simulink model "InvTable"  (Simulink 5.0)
settings: Solver=FixedStepDiscrete  StartTime=0.0  StopTime=inf  FixedStep=samplePeriod  RelTol=1e-3
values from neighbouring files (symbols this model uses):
  a0 = zeros(1, nAct)    [initialize.m]    (also in quake.m = 0; rspect.m = 1)
  azMask = zeros(nAcc, 1)    [initialize.m]
  bal = [[ 1  1  1  1  0  0  0  0  0  0  0  0]    [initialize.m]
  cmap = jet    [initialize.m]    (also in tableAnimation.m = self.cmap)
  ea_t = zeros(3, nAcc)    [initialize.m]
  faces = nAct               			+ [ 1  2  3  4    [initialize.m]    (also in tableAnimation.m = self.faces)
  flowCanon = 63090.2    [initialize.m]
  fmax = zeros(nAct, 1)    [initialize.m]
  gasConstant = 1.8    [initialize.m]
  gee = 1.0    (= 1)    [initialize.m]    (also in accelA2T.m = h(24); accelT2A.m = h(24); Test.m)
  iactParamsX = [actParamsX, dfGain, solver]    [initialize.m]
  iactParamsY = [actParamsY, dfGain, solver]    [initialize.m]
  iactParamsZ = [actParamsZ, dfGain, solver]    [initialize.m]
  inertia = [Ixx 0 0; 0 Iyy 0; 0 0 Izz]    [initialize.m]
  inertiaCanon = 0.1130    (= 0.113)    [initialize.m]
  linAccelCanon = 9800.0    (= 9800)    [initialize.m]    (also in accelA2T.m = h(19); accelT2A.m = h(19); Test.m)
  lines = nAct               			+ [ 1  2  3  4  1    				5  6  7  8  5    				9 10 11 12  9    				0  2  6 10       				0  3  7 11       				0  4  8 12  0];  	lines(find(lines==nAct)) = 0    [initialize.m]    (also in tableAnimation.m = self.lines; viewer.m = 1)
  linVelocCanon = 1000.0    (= 1000)    [initialize.m]    (also in Test.m)
  mass = [massX massY massZ]'    [initialize.m]
  massCanon = 0.4535924e-06    (= 4.535924e-07)    [initialize.m]
  maxDispl = [maxDisplX  			maxDisplY  			maxDisplZ  			maxDisplZ * linVelocCanon / rollRadius  * 180/pi  			maxDisplZ * linVelocCanon / pitchRadius * 180/pi  			min(maxDisplX, maxDisplY) * linVelocCanon / yawRadius * 180/pi]    [initialize.m]
  maxOilVolume = volume * (1 - (precharge/supplyPress)^(1/gasConstant))    (= 32.2704137442)    [initialize.m]
  maxVeloc = [maxVelocX  			maxVelocY  			maxVelocZ  			maxVelocZ * linVelocCanon / rollRadius  * 180/pi  			maxVelocZ * linVelocCanon / pitchRadius * 180/pi  			min(maxVelocX, maxVelocY) * linVelocCanon / yawRadius * 180/pi]    [initialize.m]
  minDispl = -maxDispl    [initialize.m]
  minVeloc = -maxVeloc    [initialize.m]
  nAct = size(rt_t, 2)    [initialize.m]    (also in tableAnimation.m = self.nAct)
  precharge = 2000    [initialize.m]
  pumpFlow = 1e10    (= 10000000000)    [initialize.m]
  ra_t = [  -20.0   -20.0   -92.0 -2590.0  2590.0   -62.0 -2133.0 -2133.0  2133.0  2133.0   -62.0    [initialize.m]    (also in accelA2T.m = [-h9   -h9 -h15 -h10  h10 -h14 -h12 -h12  h12  h12 -h16; accelT2A.m = [-h9   -h9 -h15 -h10  h10 -h14 -h12 -h12  h12  h12 -h16)
  rb_w = [-5692.1 -5692.1  5692.1  5692.1 -2500.0 -2500.0  2500.0  2500.0 -2400.0 -2400.0  2400.0  2400.0    [initialize.m]    (also in tableAnimation.m = rtxrb_w(:,end-nAct+1:end); positT2A.m = [-h4 -h4  h4  h4 -h1 -h1  h1  h1 -h6 -h6  h6  h6)
  returnPress = 50    [initialize.m]
  rgt = -rtg    [initialize.m]
  roll = tbl(4)    [positT2A.m]
  rotAccelCanon = 1    [initialize.m]    (also in accelA2T.m = h(22); accelT2A.m = h(22); Test.m)
  rotForceCanon = 1000    [initialize.m]    (also in forceA2T.m = h(23); Test.m)
  rotVelocCanon = 1    [initialize.m]    (also in accelA2T.m = h(21); accelT2A.m = h(21); Test.m)
  rt_t = [-3106.4 -3106.4  3106.4  3106.4 -2500.0 -2500.0  2500.0  2500.0 -2400.0 -2400.0  2400.0  2400.0    [initialize.m]    (also in positT2A.m = [rt_tx rt_ty rt_tz])
  rtg = cg    [initialize.m]
  rtx_t = [rt_t	topPlane.topLeft(:)  topPlane.topRight(:)  					topPlane.botRight(:) topPlane.botLeft(:)   					midPlane.topLeft(:)  midPlane.topRight(:)  					midPlane.botRight(:) midPlane.botLeft(:)   					botPlane.topLeft(:)  botPlane.topRight(:)  					botPlane.botRight(:) botPlane.botLeft(:)]    [initialize.m]
  samplePeriod = 1/1024    (= 0.0009765625)    [initialize.m]    (also in viewer.m = eval(getHeaderValue(header, 'DELTA_T')))
  supplyPress = 3000    [initialize.m]
  volume = 160    [initialize.m]    (also in quake.m = volume / 231.0)
  volumeCanon = 3785412.0    (= 3785412)    [initialize.m]
  zlim = [min(rb_w(3,:)) 2*halfLengthZ*lengthCanon]    [initialize.m]
undefined symbols (not defined in the file or in its folder): magnitude
libraries: aerospace x51, simulink x26, simulink_extras x1
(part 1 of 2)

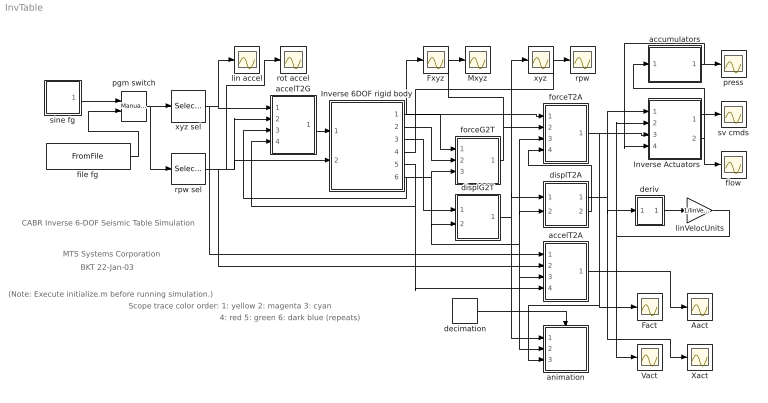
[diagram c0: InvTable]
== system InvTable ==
  note: CABR Inverse 6-DOF Seismic Table Simulation
  note: BKT 22-Jan-03
  note: MTS Systems Corporation
  note: (Note: Execute initialize.m before running simulation.)
  note: Scope trace color order: 1: yellow 2: magenta 3: cyan
  note: 4: red 5: green 6: dark blue (repeats)
  Aact : Scope
  Fact : Scope
  Fxyz : Scope
  Inverse 6DOF rigid body : Subsystem
  Inverse Actuators : Subsystem
  Mxyz : Scope
  Vact : Scope
  Xact : Scope
  accelT2A : Subsystem
  accelT2G : Subsystem
  accumulators : Subsystem
  animation : Subsystem  TreatAsAtomicUnit=on  mask{type=2, azim=-37.5, elev=15}
      mask prompts: type "Drawing type (0: none, 1: wire frame, 2: solid)"; azim "View azimuth (degrees)"; elev "View elevation (degrees)"
  decimation : DiscretePulseGenerator  Period=64  SampleTime=samplePeriod
  deriv : Subsystem  mask{T=samplePeriod}
      mask prompts: T "Sample period (sec)"
  displG2T : Subsystem
  displT2A : Subsystem
  file fg : FromFile  FileName=KobeAccel.mat  SampleTime=samplePeriod
  flow : Scope
  forceG2T : Subsystem
  forceT2A : Subsystem
  lin accel : Scope
  linVelocUnits : Gain  Gain=1/linVelocCanon
  pgm switch : simulink/Signal Routing/Manual Switch  sw=1  action=0
  press : Scope
  rot accel : Scope
  rpw : Scope
  rpw sel : Selector  Elements=[4 5 6]  InputPortWidth=6
  sine fg : Subsystem  mask(Sine Function Generator){dof=roll, ampl=200, freq=1, spanInterval=1, offset=[0 0 0 0 0 0]}
      mask prompts: ampl "Amplitude"; freq "Frequency (Hz)"; spanInterval "Span interval (sec)"
  sv cmds : Scope
  xyz : Scope
  xyz sel : Selector  Elements=[1 2 3]  InputPortWidth=6
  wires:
  xyz sel/1 -> lin accel/1, accelT2G/1(xyz), accelT2A/1(xyz)
  sine fg/1(out) -> pgm switch/1
  rpw sel/1 -> accelT2G/2(rpw), Inverse 6DOF rigid body/2(rot accel), rot accel/1, accelT2A/2(rpw)
  accelT2G/1(out) -> Inverse 6DOF rigid body/1(lin accel)
  Inverse 6DOF rigid body/1(Fxyz) -> forceG2T/1(xyz), forceT2A/1(xyz), Fxyz/1
  Inverse 6DOF rigid body/2(Mxyz) -> forceG2T/2(rpw)
  Inverse 6DOF rigid body/6(DCM) -> accelT2G/3(DCM), forceG2T/3(DCM), forceT2A/3(DCM), displT2A/2(DCM), accelT2A/3(DCM), animation/2(DCM), displG2T/2(DCM)
  forceG2T/1(out) -> forceT2A/2(rpw), Mxyz/1
  displT2A/2(dir) -> forceT2A/4(dir)
  Inverse 6DOF rigid body/3(xyz) -> displG2T/1(xyz)
  Inverse 6DOF rigid body/5(rot veloc) -> accelT2G/4(rot veloc), accelT2A/4(rot veloc)
  displG2T/1(out) -> xyz/1, displT2A/1(xyz), animation/1(xyz)
  Inverse 6DOF rigid body/4(rpw) -> rpw/1
  deriv/1(out) -> linVelocUnits/1
  forceT2A/1(out) -> Inverse Actuators/3(force), Fact/1, animation/3(Fact)
  Inverse Actuators/1(cmd) -> sv cmds/1
  Inverse Actuators/2(flow) -> flow/1, accumulators/1(flow)
  accumulators/1(press) -> Inverse Actuators/4(press), press/1
  displT2A/1(out) -> Inverse Actuators/1(displ), Xact/1, deriv/1(inp)
  linVelocUnits/1 -> Inverse Actuators/2(veloc), Vact/1
  pgm switch/1 -> rpw sel/1, xyz sel/1
  file fg/1 -> pgm switch/2
  accelT2A/1(out) -> Aact/1
  decimation/1 -> animation/Trigger

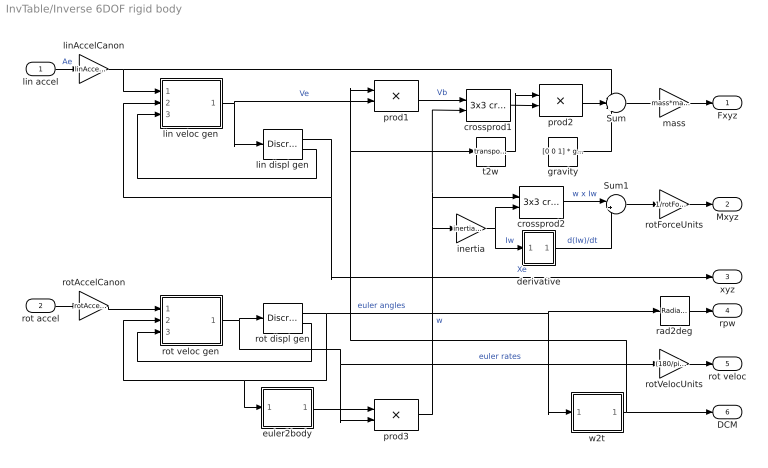
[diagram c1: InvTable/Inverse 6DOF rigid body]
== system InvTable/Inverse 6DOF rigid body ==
  lin accel : Inport
  rot accel : Inport  Port=2
  Sum : Sum  Inputs=+-+
  Sum1 : Sum  Inputs=|++
  crossprod1 : aerospace/Axes Transformations/3x3 cross product
  crossprod2 : aerospace/Axes Transformations/3x3 cross product
  derivative : Subsystem  mask{T=samplePeriod}
      mask prompts: T "Sample period (sec)"
  euler2body : Subsystem
  gravity : Constant  Value=[0 0 1] * gee * linAccelCanon * ~static
  inertia : Gain  Gain=inertia*inertiaCanon  Multiplication=Matrix(K*u)
  lin displ gen : DiscreteIntegrator  IntegratorMethod=Backward Euler  LimitOutput=on  UpperSaturationLimit=maxDispl(1:3)  LowerSaturationLimit=minDispl(1:3)  ShowSaturationPort=on  SampleTime=-1
  lin veloc gen : Subsystem  mask{maxVeloc=maxVeloc(1:3)*linVelocCanon, minVeloc=minVeloc(1:3)*linVelocCanon, maxDispl=maxDispl(1:3), minDispl=minDispl(1:3)}
      mask prompts: maxVeloc "Max velocity"; minVeloc "Min velocity"; maxDispl "Max displacement"; minDispl "Min displacement"
  linAccelCanon : Gain  Gain=linAccelCanon
  mass : Gain  Gain=mass*massCanon
  prod1 : Product  Multiplication=Matrix(*)
  prod2 : Product  Multiplication=Matrix(*)
  prod3 : Product  Multiplication=Matrix(*)
  rad2deg : simulink_extras/Transformations/Radians to Degrees
  rot displ gen : DiscreteIntegrator  LimitOutput=on  UpperSaturationLimit=maxDispl(4:6)*pi/180  LowerSaturationLimit=minDispl(4:6)*pi/180  ShowSaturationPort=on  SampleTime=-1
  rot veloc gen : Subsystem  mask{maxVeloc=maxVeloc(4:6)*rotVelocCanon*pi/180, minVeloc=minVeloc(4:6)*rotVelocCanon*pi/180, maxDispl=maxDispl(4:6)*pi/180, minDispl=minDispl(4:6)*pi/180}
      mask prompts: maxVeloc "Max velocity"; minVeloc "Min velocity"; maxDispl "Max displacement"; minDispl "Min displacement"
  rotAccelCanon : Gain  Gain=rotAccelCanon*(pi/180)
  rotForceUnits : Gain  Gain=1/rotForceCanon
  rotVelocUnits : Gain  Gain=(180/pi)/rotVelocCanon
  t2w : Math  Operator=transpose
  w2t : Subsystem
  Fxyz : Outport
  Mxyz : Outport  Port=2
  xyz : Outport  Port=3
  rpw : Outport  Port=4
  rot veloc : Outport  Port=5
  DCM : Outport  Port=6
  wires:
  lin accel/1 -> linAccelCanon/1  "Ae"
  lin veloc gen/1(veloc) -> prod1/2, lin displ gen/1  "Ve"
  Sum/1 -> mass/1
  gravity/1 -> Sum/3
  rot accel/1 -> rotAccelCanon/1
  inertia/1 -> crossprod2/2, derivative/1(inp)  "Iw"
  crossprod2/1 -> Sum1/1  "w x Iw"
  derivative/1(out) -> Sum1/2  "d(Iw)/dt"
  Sum1/1 -> rotForceUnits/1
  lin displ gen/1 -> xyz/1, lin veloc gen/2(displ)  "Xe"
  prod1/1 -> crossprod1/1  "Vb"
  mass/1 -> Fxyz/1
  crossprod1/1 -> prod2/2
  t2w/1 -> prod2/1
  prod2/1 -> Sum/2
  rotAccelCanon/1 -> rot veloc gen/1(accel)
  rad2deg/1 -> rpw/1
  rotVelocUnits/1 -> rot veloc/1
  linAccelCanon/1 -> Sum/1, lin veloc gen/1(accel)
  rotForceUnits/1 -> Mxyz/1
  euler2body/1(out) -> prod3/1
  w2t/1(DCM) -> DCM/1, prod1/1, t2w/1
  rot veloc gen/1(veloc) -> rot displ gen/1, prod3/2, rotVelocUnits/1  "euler rates"
  prod3/1 -> inertia/1, crossprod1/2, crossprod2/1  "w"
  rot displ gen/1 -> rad2deg/1, w2t/1(rpw), euler2body/1(rpw), rot veloc gen/2(displ)  "euler angles"
  lin displ gen/2 -> lin veloc gen/3(reset)
  rot displ gen/2 -> rot veloc gen/3(reset)

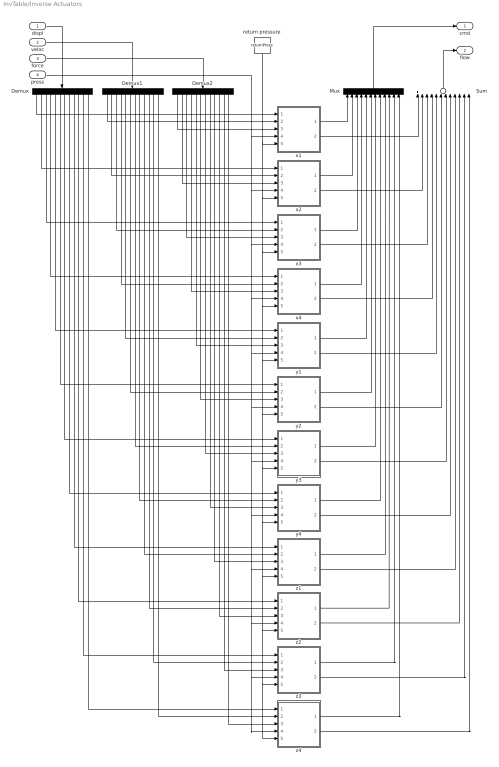
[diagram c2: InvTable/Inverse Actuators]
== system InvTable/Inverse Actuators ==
  displ : Inport
  veloc : Inport  Port=2
  force : Inport  Port=3
  press : Inport  Port=4
  Demux : Demux  Orientation=down  Outputs=12
  Demux1 : Demux  Orientation=down  Outputs=12
  Demux2 : Demux  Orientation=down  Outputs=12
  Mux : Mux  Orientation=up  Inputs=12
  Sum : Sum  Orientation=up  Inputs=12
  return pressure : Constant  Orientation=down  Value=returnPress
  x1 : Subsystem  mask(Inverse Actuator){params=iactParamsX}
      mask prompts: params "Parameter vector"
  x2 : Subsystem  mask(Inverse Actuator){params=iactParamsX}
      mask prompts: params "Parameter vector"
  x3 : Subsystem  mask(Inverse Actuator){params=iactParamsX}
      mask prompts: params "Parameter vector"
  x4 : Subsystem  mask(Inverse Actuator){params=iactParamsX}
      mask prompts: params "Parameter vector"
  y1 : Subsystem  mask(Inverse Actuator){params=iactParamsY}
      mask prompts: params "Parameter vector"
  y2 : Subsystem  mask(Inverse Actuator){params=iactParamsY}
      mask prompts: params "Parameter vector"
  y3 : Subsystem  mask(Inverse Actuator){params=iactParamsY}
      mask prompts: params "Parameter vector"
  y4 : Subsystem  mask(Inverse Actuator){params=iactParamsY}
      mask prompts: params "Parameter vector"
  z1 : Subsystem  mask(Inverse Actuator){params=iactParamsZ}
      mask prompts: params "Parameter vector"
  z2 : Subsystem  mask(Inverse Actuator){params=iactParamsZ}
      mask prompts: params "Parameter vector"
  z3 : Subsystem  mask(Inverse Actuator){params=iactParamsZ}
      mask prompts: params "Parameter vector"
  z4 : Subsystem  mask(Inverse Actuator){params=iactParamsZ}
      mask prompts: params "Parameter vector"
  cmd : Outport
  flow : Outport  Port=2
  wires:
  displ/1 -> Demux/1
  veloc/1 -> Demux1/1
  Demux/1 -> x1/1(displ)
  Demux/2 -> x2/1(displ)
  Demux1/1 -> x1/2(veloc)
  Demux2/1 -> x1/3(force)
  Demux1/2 -> x2/2(veloc)
  Demux2/2 -> x2/3(force)
  Demux/3 -> x3/1(displ)
  Demux1/3 -> x3/2(veloc)
  Demux2/3 -> x3/3(force)
  Demux/4 -> x4/1(displ)
  Demux1/4 -> x4/2(veloc)
  Demux2/4 -> x4/3(force)
  Demux/5 -> y1/1(displ)
  Demux1/5 -> y1/2(veloc)
  Demux2/5 -> y1/3(force)
  Demux/6 -> y2/1(displ)
  Demux1/6 -> y2/2(veloc)
  Demux2/6 -> y2/3(force)
  Demux/7 -> y3/1(displ)
  Demux1/7 -> y3/2(veloc)
  Demux2/7 -> y3/3(force)
  Demux/8 -> y4/1(displ)
  Demux1/8 -> y4/2(veloc)
  Demux2/8 -> y4/3(force)
  x3/1(cmd) -> Mux/3
  x4/1(cmd) -> Mux/4
  Mux/1 -> cmd/1
  y1/1(cmd) -> Mux/5
  y2/1(cmd) -> Mux/6
  y3/1(cmd) -> Mux/7
  y4/1(cmd) -> Mux/8
  force/1 -> Demux2/1
  x1/1(cmd) -> Mux/1
  x2/1(cmd) -> Mux/2
  x1/2(flow) -> Sum/1
  x2/2(flow) -> Sum/2
  x3/2(flow) -> Sum/3
  x4/2(flow) -> Sum/4
  y1/2(flow) -> Sum/5
  y2/2(flow) -> Sum/6
  y3/2(flow) -> Sum/7
  y4/2(flow) -> Sum/8
  Sum/1 -> flow/1
  press/1 -> z3/4(spl press), z4/4(spl press), z2/4(spl press), z1/4(spl press), y4/4(spl press), y3/4(spl press), y2/4(spl press), y1/4(spl press), x4/4(spl press), x3/4(spl press), x2/4(spl press), x1/4(spl press)
  return pressure/1 -> z3/5(rtn press), z4/5(rtn press), z2/5(rtn press), z1/5(rtn press), y4/5(rtn press), y3/5(rtn press), y2/5(rtn press), y1/5(rtn press), x4/5(rtn press), x3/5(rtn press), x2/5(rtn press), x1/5(rtn press)
  Demux/9 -> z1/1(displ)
  Demux/10 -> z2/1(displ)
  Demux/11 -> z3/1(displ)
  Demux1/9 -> z1/2(veloc)
  Demux/12 -> z4/1(displ)
  Demux1/10 -> z2/2(veloc)
  Demux1/11 -> z3/2(veloc)
  Demux1/12 -> z4/2(veloc)
  Demux2/9 -> z1/3(force)
  Demux2/10 -> z2/3(force)
  Demux2/12 -> z4/3(force)
  Demux2/11 -> z3/3(force)
  z1/1(cmd) -> Mux/9
  z2/1(cmd) -> Mux/10
  z3/1(cmd) -> Mux/11
  z4/1(cmd) -> Mux/12
  z1/2(flow) -> Sum/9
  z2/2(flow) -> Sum/10
  z3/2(flow) -> Sum/11
  z4/2(flow) -> Sum/12

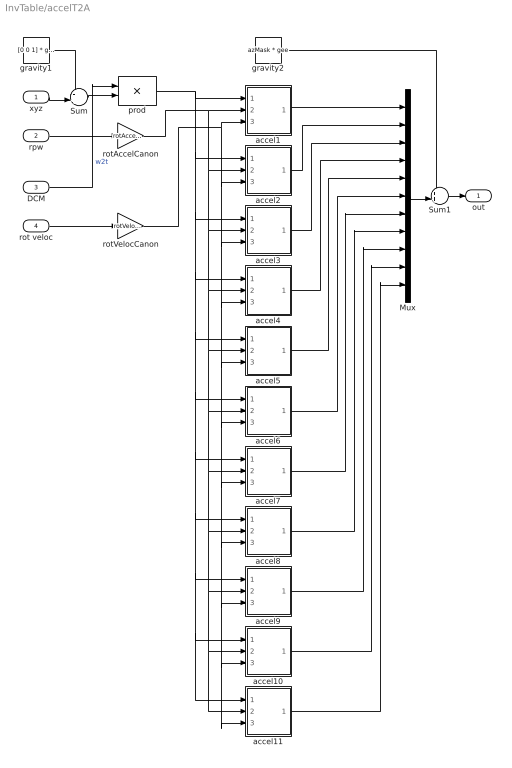
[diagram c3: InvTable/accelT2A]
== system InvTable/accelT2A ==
  xyz : Inport
  rpw : Inport  Port=2
  DCM : Inport  Port=3
  rot veloc : Inport  Port=4
  Mux : Mux  Inputs=11
  Sum : Sum  Inputs=-+|
  Sum1 : Sum  Inputs=++|
  accel1 : Subsystem  mask{id=1}
      mask prompts: id "Accelerometer number"
  accel10 : Subsystem  mask{id=10}
      mask prompts: id "Accelerometer number"
  accel11 : Subsystem  mask{id=11}
      mask prompts: id "Accelerometer number"
  accel2 : Subsystem  mask{id=2}
      mask prompts: id "Accelerometer number"
  accel3 : Subsystem  mask{id=3}
      mask prompts: id "Accelerometer number"
  accel4 : Subsystem  mask{id=4}
      mask prompts: id "Accelerometer number"
  accel5 : Subsystem  mask{id=5}
      mask prompts: id "Accelerometer number"
  accel6 : Subsystem  mask{id=6}
      mask prompts: id "Accelerometer number"
  accel7 : Subsystem  mask{id=7}
      mask prompts: id "Accelerometer number"
  accel8 : Subsystem  mask{id=8}
      mask prompts: id "Accelerometer number"
  accel9 : Subsystem  mask{id=9}
      mask prompts: id "Accelerometer number"
  gravity1 : Constant  Value=[0 0 1] * gee
  gravity2 : Constant  Value=azMask * gee
  prod : Product  Multiplication=Matrix(*)
  rotAccelCanon : Gain  Gain=rotAccelCanon*(pi/180)/linAccelCanon
  rotVelocCanon : Gain  Gain=rotVelocCanon*(pi/180)/sqrt(linAccelCanon)
  out : Outport
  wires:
  gravity2/1 -> Sum1/1
  Sum1/1 -> out/1
  Mux/1 -> Sum1/2
  accel7/1(out) -> Mux/7
  accel8/1(out) -> Mux/8
  accel9/1(out) -> Mux/9
  accel10/1(out) -> Mux/10
  accel11/1(out) -> Mux/11
  gravity1/1 -> Sum/1
  xyz/1 -> Sum/2
  Sum/1 -> prod/2
  accel3/1(out) -> Mux/3
  accel4/1(out) -> Mux/4
  accel5/1(out) -> Mux/5
  accel6/1(out) -> Mux/6
  accel2/1(out) -> Mux/2
  accel1/1(out) -> Mux/1
  rotAccelCanon/1 -> accel1/2(rotacc), accel2/2(rotacc), accel3/2(rotacc), accel4/2(rotacc), accel5/2(rotacc), accel6/2(rotacc), accel7/2(rotacc), accel8/2(rotacc), accel9/2(rotacc), accel11/2(rotacc), accel10/2(rotacc)
  rotVelocCanon/1 -> accel1/3(rotvel), accel2/3(rotvel), accel3/3(rotvel), accel4/3(rotvel), accel5/3(rotvel), accel6/3(rotvel), accel7/3(rotvel), accel8/3(rotvel), accel9/3(rotvel), accel11/3(rotvel), accel10/3(rotvel)
  DCM/1 -> prod/1  "w2t"
  rot veloc/1 -> rotVelocCanon/1
  rpw/1 -> rotAccelCanon/1
  prod/1 -> accel1/1(linacc), accel2/1(linacc), accel3/1(linacc), accel4/1(linacc), accel5/1(linacc), accel6/1(linacc), accel7/1(linacc), accel8/1(linacc), accel9/1(linacc), accel11/1(linacc), accel10/1(linacc)

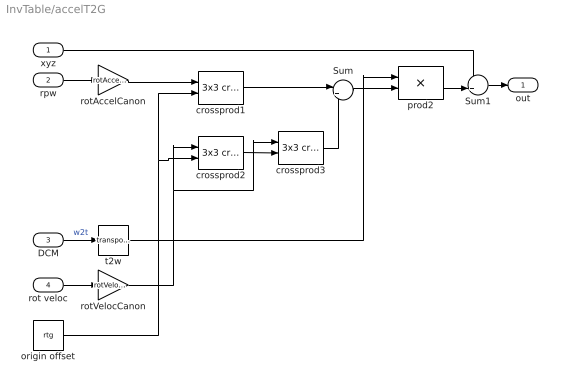
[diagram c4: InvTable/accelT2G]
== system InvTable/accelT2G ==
  xyz : Inport
  rpw : Inport  Port=2
  DCM : Inport  Port=3
  rot veloc : Inport  Port=4
  Sum : Sum  Inputs=|++
  Sum1 : Sum  Inputs=++|
  crossprod1 : aerospace/Axes Transformations/3x3 cross product
  crossprod2 : aerospace/Axes Transformations/3x3 cross product
  crossprod3 : aerospace/Axes Transformations/3x3 cross product
  origin offset : Constant  Value=rtg
  prod2 : Product  Multiplication=Matrix(*)
  rotAccelCanon : Gain  Gain=rotAccelCanon*(pi/180)/linAccelCanon
  rotVelocCanon : Gain  Gain=rotVelocCanon*(pi/180)/sqrt(linAccelCanon)
  t2w : Math  Operator=transpose
  out : Outport
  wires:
  crossprod1/1 -> Sum/1
  crossprod3/1 -> Sum/2
  Sum1/1 -> out/1
  prod2/1 -> Sum1/2
  crossprod2/1 -> crossprod3/2
  Sum/1 -> prod2/2
  origin offset/1 -> crossprod1/2, crossprod2/2
  rotAccelCanon/1 -> crossprod1/1
  rpw/1 -> rotAccelCanon/1
  t2w/1 -> prod2/1
  xyz/1 -> Sum1/1
  rot veloc/1 -> rotVelocCanon/1
  DCM/1 -> t2w/1  "w2t"
  rotVelocCanon/1 -> crossprod3/1, crossprod2/1

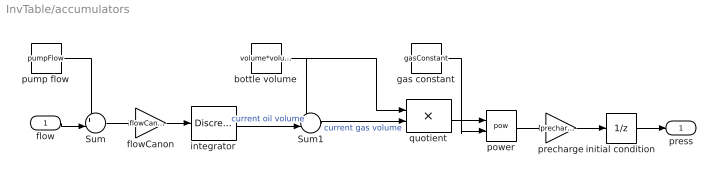
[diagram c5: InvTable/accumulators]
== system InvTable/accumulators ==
  flow : Inport
  Sum : Sum  Inputs=+-|
  Sum1 : Sum  Inputs=+-|
  bottle volume : Constant  Value=volume*volumeCanon
  flowCanon : Gain  Gain=flowCanon
  gas constant : Constant  Value=gasConstant
  initial condition : UnitDelay  X0=supplyPress  SampleTime=-1
  integrator : DiscreteIntegrator  InitialCondition=maxOilVolume*volumeCanon  LimitOutput=on  UpperSaturationLimit=maxOilVolume*volumeCanon  LowerSaturationLimit=0  SampleTime=-1
  power : Math  Operator=pow
  precharge : Gain  Gain=precharge
  pump flow : Constant  Value=pumpFlow
  quotient : Product  Inputs=*/
  press : Outport
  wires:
  initial condition/1 -> press/1
  flowCanon/1 -> integrator/1
  flow/1 -> Sum/2
  integrator/1 -> Sum1/2  "current oil volume"
  quotient/1 -> power/1
  Sum1/1 -> quotient/2  "current gas volume"
  precharge/1 -> initial condition/1
  power/1 -> precharge/1
  gas constant/1 -> power/2
  bottle volume/1 -> quotient/1, Sum1/1
  Sum/1 -> flowCanon/1
  pump flow/1 -> Sum/1

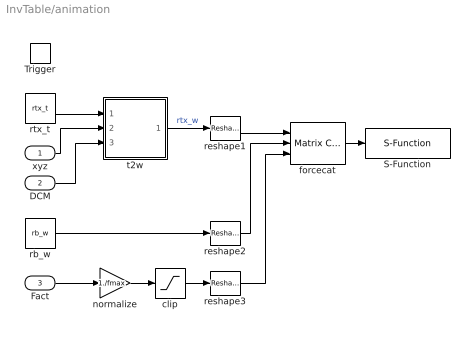
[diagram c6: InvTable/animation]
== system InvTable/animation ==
  xyz : Inport
  DCM : Inport  Port=2
  Fact : Inport  Port=3
  Trigger : TriggerPort
  S-Function : S-Function  FunctionName=tableAnimation  Parameters=type,azim,elev,nAct,zlim,lines,faces,cmap
  clip : Saturate  UpperLimit=1  LowerLimit=-1
  forcecat : simulink/Math Operations/Matrix Concatenation  numInports=3  catMethod=Vertical
  normalize : Gain  Gain=1./fmax
  rb_w : Constant  Value=rb_w
  reshape1 : simulink/Math Operations/Reshape  OutputDimensionality=1-D array  OutputDimensions=[1,1]
  reshape2 : simulink/Math Operations/Reshape  OutputDimensionality=1-D array  OutputDimensions=[1,1]
  reshape3 : simulink/Math Operations/Reshape  OutputDimensionality=1-D array  OutputDimensions=[1,1]
  rtx_t : Constant  Value=rtx_t
  t2w : Subsystem
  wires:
  DCM/1 -> t2w/3(DCM)
  xyz/1 -> t2w/2(xyz)
  rtx_t/1 -> t2w/1(inp)
  reshape3/1 -> forcecat/3
  reshape2/1 -> forcecat/2
  rb_w/1 -> reshape2/1
  forcecat/1 -> S-Function/1
  reshape1/1 -> forcecat/1
  Fact/1 -> normalize/1
  t2w/1(out) -> reshape1/1  "rtx_w"
  normalize/1 -> clip/1
  clip/1 -> reshape3/1

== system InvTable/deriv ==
  inp : Inport
  1/T : Gain  Gain=1/T
  Sum : Sum  Inputs=|+-
  Unit Delay : UnitDelay  SampleTime=-1
  out : Outport
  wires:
  inp/1 -> Sum/1, Unit Delay/1
  Unit Delay/1 -> Sum/2
  Sum/1 -> 1/T/1
  1/T/1 -> out/1

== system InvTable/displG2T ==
  xyz : Inport
  DCM : Inport  Port=2
  Sum1 : Sum  Inputs=++-
  origin offset : Constant  Value=rgt
  prod : Product  Multiplication=Matrix(*)
  t2w : Math  Operator=transpose
  out : Outport
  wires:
  t2w/1 -> prod/1
  DCM/1 -> t2w/1
  origin offset/1 -> prod/2, Sum1/3
  xyz/1 -> Sum1/1
  prod/1 -> Sum1/2
  Sum1/1 -> out/1

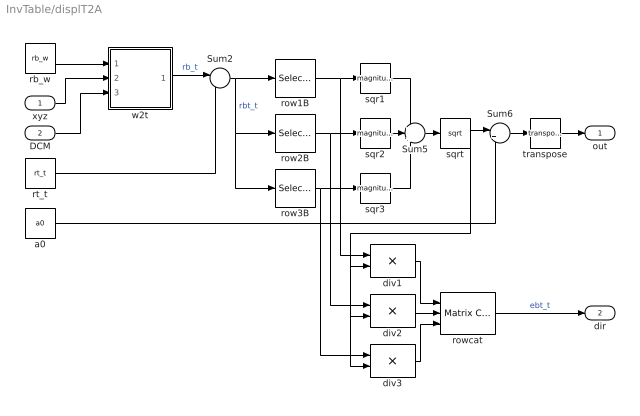
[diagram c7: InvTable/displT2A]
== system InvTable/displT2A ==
  xyz : Inport
  DCM : Inport  Port=2
  Sum2 : Sum  Inputs=|-+
  Sum5 : Sum  Inputs=+++
  Sum6 : Sum  Inputs=|+-
  a0 : Constant  Value=a0
  div1 : Product  Inputs=*/
  div2 : Product  Inputs=*/
  div3 : Product  Inputs=*/
  rb_w : Constant  Value=rb_w
  row1B : Selector  InputType=Matrix  Elements=[1 3]  Columns=-1  InputPortWidth=3
  row2B : Selector  InputType=Matrix  Elements=[1 3]  Rows=2  Columns=-1  InputPortWidth=3
  row3B : Selector  InputType=Matrix  Elements=[1 3]  Rows=3  Columns=-1  InputPortWidth=3
  rowcat : simulink/Math Operations/Matrix Concatenation  numInports=3  catMethod=Vertical
  rt_t : Constant  Value=rt_t
  sqr1 : Math  Operator=magnitude^2
  sqr2 : Math  Operator=magnitude^2
  sqr3 : Math  Operator=magnitude^2
  sqrt : Math  Operator=sqrt
  transpose : Math  Operator=transpose
  w2t : Subsystem
  out : Outport
  dir : Outport  Port=2
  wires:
  xyz/1 -> w2t/2(xyz)
  rb_w/1 -> w2t/1(inp)
  rt_t/1 -> Sum2/2
  row2B/1 -> sqr2/1, div2/1
  row1B/1 -> sqr1/1, div1/1
  row3B/1 -> sqr3/1, div3/1
  Sum5/1 -> sqrt/1
  a0/1 -> Sum6/2
  sqrt/1 -> Sum6/1, div1/2, div2/2, div3/2
  w2t/1(out) -> Sum2/1  "rb_t"
  Sum2/1 -> row3B/1, row2B/1, row1B/1  "rbt_t"
  sqr1/1 -> Sum5/1
  sqr2/1 -> Sum5/2
  sqr3/1 -> Sum5/3
  rowcat/1 -> dir/1  "ebt_t"
  div1/1 -> rowcat/1
  div2/1 -> rowcat/2
  div3/1 -> rowcat/3
  DCM/1 -> w2t/3(DCM)
  Sum6/1 -> transpose/1
  transpose/1 -> out/1

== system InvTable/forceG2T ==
  xyz : Inport
  rpw : Inport  Port=2
  DCM : Inport  Port=3
  Sum : Sum  Inputs=-+|
  crossprod : aerospace/Axes Transformations/3x3 cross product
  origin offset : Constant  Value=rtg
  prod : Product  Multiplication=Matrix(*)
  rotForceUnits : Gain  Gain=1/rotForceCanon
  out : Outport
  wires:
  origin offset/1 -> crossprod/2
  prod/1 -> crossprod/1
  DCM/1 -> prod/1
  xyz/1 -> prod/2
  rotForceUnits/1 -> Sum/1
  crossprod/1 -> rotForceUnits/1
  Sum/1 -> out/1
  rpw/1 -> Sum/2

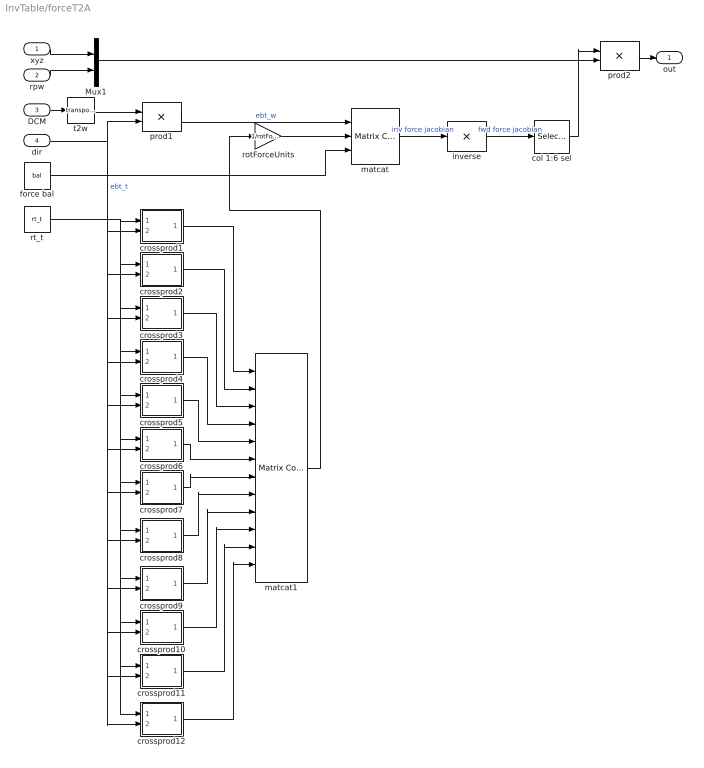
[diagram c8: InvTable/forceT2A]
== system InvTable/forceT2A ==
  xyz : Inport
  rpw : Inport  Port=2
  DCM : Inport  Port=3
  dir : Inport  Port=4
  Mux1 : Mux  Inputs=2
  col 1:6 sel : Selector  InputType=Matrix  Elements=[1 2 3 4 ]  Rows=-1  Columns=1:6
  crossprod1 : Subsystem  mask{id=1}
      mask prompts: id "Actuator number"
  crossprod10 : Subsystem  mask{id=10}
      mask prompts: id "Actuator number"
  crossprod11 : Subsystem  mask{id=11}
      mask prompts: id "Actuator number"
  crossprod12 : Subsystem  mask{id=12}
      mask prompts: id "Actuator number"
  crossprod2 : Subsystem  mask{id=2}
      mask prompts: id "Actuator number"
  crossprod3 : Subsystem  mask{id=3}
      mask prompts: id "Actuator number"
  crossprod4 : Subsystem  mask{id=4}
      mask prompts: id "Actuator number"
  crossprod5 : Subsystem  mask{id=5}
      mask prompts: id "Actuator number"
  crossprod6 : Subsystem  mask{id=6}
      mask prompts: id "Actuator number"
  crossprod7 : Subsystem  mask{id=7}
      mask prompts: id "Actuator number"
  crossprod8 : Subsystem  mask{id=8}
      mask prompts: id "Actuator number"
  crossprod9 : Subsystem  mask{id=9}
      mask prompts: id "Actuator number"
  force bal : Constant  Value=bal
  inverse : Product  Inputs=/  Multiplication=Matrix(*)
  matcat : simulink/Math Operations/Matrix Concatenation  numInports=3  catMethod=Vertical
  matcat1 : simulink/Math Operations/Matrix Concatenation  numInports=12  catMethod=Horizontal
  prod1 : Product  Multiplication=Matrix(*)
  prod2 : Product  Multiplication=Matrix(*)
  rotForceUnits : Gain  Gain=1/rotForceCanon
  rt_t : Constant  Value=rt_t
  t2w : Math  Operator=transpose
  out : Outport
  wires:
  force bal/1 -> matcat/3
  t2w/1 -> prod1/1
  crossprod8/1(AxB) -> matcat1/8
  crossprod7/1(AxB) -> matcat1/7
  crossprod6/1(AxB) -> matcat1/6
  crossprod5/1(AxB) -> matcat1/5
  crossprod4/1(AxB) -> matcat1/4
  crossprod3/1(AxB) -> matcat1/3
  crossprod2/1(AxB) -> matcat1/2
  crossprod1/1(AxB) -> matcat1/1
  matcat1/1 -> rotForceUnits/1
  rt_t/1 -> crossprod2/1(A), crossprod3/1(A), crossprod4/1(A), crossprod5/1(A), crossprod6/1(A), crossprod7/1(A), crossprod8/1(A), crossprod9/1(A), crossprod10/1(A), crossprod12/1(A), crossprod11/1(A), crossprod1/1(A)
  prod1/1 -> matcat/1  "ebt_w"
  dir/1 -> crossprod2/2(B), crossprod3/2(B), crossprod4/2(B), crossprod5/2(B), crossprod6/2(B), crossprod7/2(B), crossprod8/2(B), crossprod12/2(B), crossprod11/2(B), crossprod10/2(B), crossprod9/2(B), crossprod1/2(B), prod1/2  "ebt_t"
  DCM/1 -> t2w/1
  matcat/1 -> inverse/1  "inv force jacobian"
  rotForceUnits/1 -> matcat/2
  prod2/1 -> out/1
  xyz/1 -> Mux1/1
  rpw/1 -> Mux1/2
  Mux1/1 -> prod2/2
  inverse/1 -> col 1:6 sel/1  "fwd force jacobian"
  col 1:6 sel/1 -> prod2/1
  crossprod9/1(AxB) -> matcat1/9
  crossprod10/1(AxB) -> matcat1/10
  crossprod11/1(AxB) -> matcat1/11
  crossprod12/1(AxB) -> matcat1/12

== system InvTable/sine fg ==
  Product : Product
  Ramp : simulink/Sources/Ramp  slope=1/spanInterval  start=0  X0=0
  Reshape : simulink/Math Operations/Reshape  OutputDimensionality=1-D array  OutputDimensions=[1,1]
  Saturation : Saturate  UpperLimit=1  LowerLimit=0
  Sum : Sum  Inputs=|++
  Zero-Order Hold : ZeroOrderHold  SampleTime=samplePeriod
  dof : Constant  Value=[7-dof : 12-dof]
  dof sel : Selector  ElementSrc=External  Elements=-1  InputPortWidth=11
  offset : Constant  Value=offset
  rowcat : simulink/Math Operations/Matrix Concatenation  numInports=3  catMethod=Vertical
  sine : Sin  Amplitude=ampl  Frequency=2 * pi * freq  SampleTime=samplePeriod
  zeros : Constant  Value=[0 0 0 0 0]'
  out : Outport
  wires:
  rowcat/1 -> dof sel/1
  zeros/1 -> rowcat/1, rowcat/3
  sine/1 -> rowcat/2
  dof/1 -> dof sel/2
  dof sel/1 -> Product/1
  Ramp/1 -> Zero-Order Hold/1
  Zero-Order Hold/1 -> Saturation/1
  Saturation/1 -> Product/2
  Reshape/1 -> out/1
  Product/1 -> Sum/1
  Sum/1 -> Reshape/1
  offset/1 -> Sum/2

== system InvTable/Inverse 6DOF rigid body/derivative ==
  inp : Inport
  1/T : Gain  Gain=1/T
  Sum : Sum  Inputs=|+-
  Unit Delay : UnitDelay  SampleTime=-1
  out : Outport
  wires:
  inp/1 -> Sum/1, Unit Delay/1
  Unit Delay/1 -> Sum/2
  Sum/1 -> 1/T/1
  1/T/1 -> out/1

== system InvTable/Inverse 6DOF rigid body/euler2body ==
  rpw : Inport
  11 : Fcn  Expr=cos(u[2])
  12 : Fcn  Expr=0
  13 : Fcn  Expr=cos(u[1])*sin(u[2])
  21 : Fcn  Expr=0
  22 : Fcn  Expr=1
  23 : Fcn  Expr=-sin(u[1])
  31 : Fcn  Expr=-sin(u[2])
  32 : Fcn  Expr=0
  33 : Fcn  Expr=cos(u[1])*cos(u[2])
  9x1->3x3 : simulink/Math Operations/Reshape  OutputDimensionality=Customize  OutputDimensions=[3,3]
  Mux2 : Mux  Orientation=down  Inputs=9
  out : Outport
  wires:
  33/1 -> Mux2/9
  23/1 -> Mux2/8
  13/1 -> Mux2/7
  Mux2/1 -> 9x1->3x3/1
  32/1 -> Mux2/6
  22/1 -> Mux2/5
  12/1 -> Mux2/4
  rpw/1 -> 13/1, 23/1, 33/1, 12/1, 22/1, 32/1, 11/1, 21/1, 31/1
  31/1 -> Mux2/3
  21/1 -> Mux2/2
  11/1 -> Mux2/1
  9x1->3x3/1 -> out/1

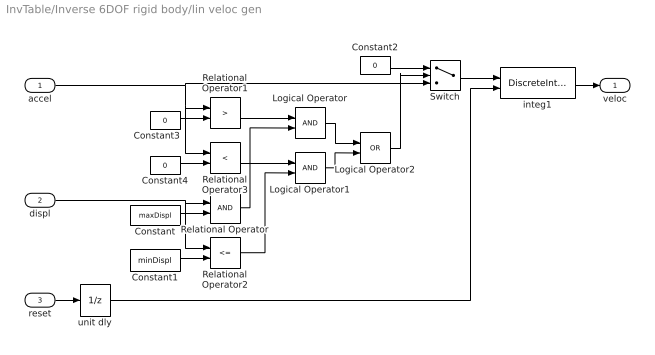
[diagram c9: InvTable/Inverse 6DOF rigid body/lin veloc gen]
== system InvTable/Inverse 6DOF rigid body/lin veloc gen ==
  accel : Inport
  displ : Inport  Port=2
  reset : Inport  Port=3
  Constant : Constant  Value=maxDispl
  Constant1 : Constant  Value=minDispl
  Constant2 : Constant  Value=0
  Constant3 : Constant  Value=0
  Constant4 : Constant  Value=0
  Logical Operator : Logic
  Logical Operator1 : Logic
  Logical Operator2 : Logic  Operator=OR
  Relational Operator : RelationalOperator
  Relational Operator1 : RelationalOperator  Operator=>
  Relational Operator2 : RelationalOperator  Operator=<=
  Relational Operator3 : RelationalOperator  Operator=<
  Switch : Switch  Threshold=0.5
  integ1 : DiscreteIntegrator  ExternalReset=either  LimitOutput=on  UpperSaturationLimit=maxVeloc  LowerSaturationLimit=minVeloc  SampleTime=-1
  unit dly : UnitDelay  SampleTime=-1
  veloc : Outport
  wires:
  reset/1 -> unit dly/1
  displ/1 -> Relational Operator2/1, Relational Operator/1
  Logical Operator1/1 -> Logical Operator2/2
  unit dly/1 -> integ1/2
  Switch/1 -> integ1/1
  Logical Operator2/1 -> Switch/2
  Constant2/1 -> Switch/1
  Logical Operator/1 -> Logical Operator2/1
  Relational Operator3/1 -> Logical Operator1/1
  Constant4/1 -> Relational Operator3/2
  Relational Operator1/1 -> Logical Operator/1
  Constant3/1 -> Relational Operator1/2
  accel/1 -> Switch/3, Relational Operator1/1, Relational Operator3/1
  Constant1/1 -> Relational Operator2/2
  Relational Operator2/1 -> Logical Operator1/2
  Relational Operator/1 -> Logical Operator/2
  Constant/1 -> Relational Operator/2
  integ1/1 -> veloc/1

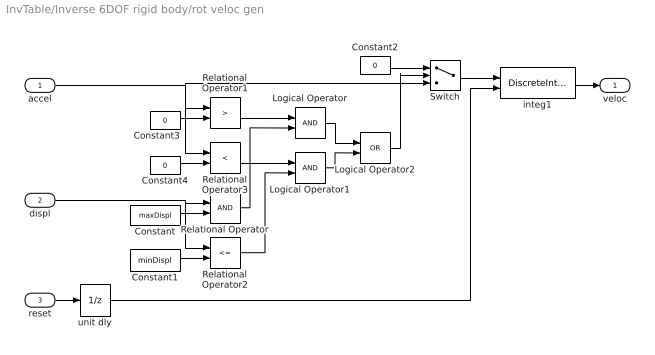
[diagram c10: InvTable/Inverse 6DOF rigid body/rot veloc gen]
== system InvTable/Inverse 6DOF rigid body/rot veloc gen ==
  accel : Inport
  displ : Inport  Port=2
  reset : Inport  Port=3
  Constant : Constant  Value=maxDispl
  Constant1 : Constant  Value=minDispl
  Constant2 : Constant  Value=0
  Constant3 : Constant  Value=0
  Constant4 : Constant  Value=0
  Logical Operator : Logic
  Logical Operator1 : Logic
  Logical Operator2 : Logic  Operator=OR
  Relational Operator : RelationalOperator
  Relational Operator1 : RelationalOperator  Operator=>
  Relational Operator2 : RelationalOperator  Operator=<=
  Relational Operator3 : RelationalOperator  Operator=<
  Switch : Switch  Threshold=0.5
  integ1 : DiscreteIntegrator  ExternalReset=either  LimitOutput=on  UpperSaturationLimit=maxVeloc  LowerSaturationLimit=minVeloc  SampleTime=-1
  unit dly : UnitDelay  SampleTime=-1
  veloc : Outport
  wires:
  integ1/1 -> veloc/1
  Constant/1 -> Relational Operator/2
  Relational Operator/1 -> Logical Operator/2
  Relational Operator2/1 -> Logical Operator1/2
  Constant1/1 -> Relational Operator2/2
  accel/1 -> Relational Operator3/1, Relational Operator1/1, Switch/3
  Constant3/1 -> Relational Operator1/2
  Relational Operator1/1 -> Logical Operator/1
  Constant4/1 -> Relational Operator3/2
  Relational Operator3/1 -> Logical Operator1/1
  Logical Operator/1 -> Logical Operator2/1
  Constant2/1 -> Switch/1
  Logical Operator2/1 -> Switch/2
  Switch/1 -> integ1/1
  unit dly/1 -> integ1/2
  Logical Operator1/1 -> Logical Operator2/2
  displ/1 -> Relational Operator/1, Relational Operator2/1
  reset/1 -> unit dly/1

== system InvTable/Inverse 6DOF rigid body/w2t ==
  rpw : Inport
  11 : Fcn  Expr=cos(u[3])*cos(u[2])-sin(u[3])*sin(u[1])*sin(u[2])
  12 : Fcn  Expr=sin(u[3])*cos(u[2])+cos(u[3])*sin(u[1])*sin(u[2])
  13 : Fcn  Expr=-cos(u[1])*sin(u[2])
  21 : Fcn  Expr=-sin(u[3])*cos(u[1])
  22 : Fcn  Expr=cos(u[3])*cos(u[1])
  23 : Fcn
  31 : Fcn  Expr=cos(u[3])*sin(u[2])+sin(u[3])*sin(u[1])*cos(u[2])
  32 : Fcn  Expr=sin(u[3])*sin(u[2])-cos(u[3])*sin(u[1])*cos(u[2])
  33 : Fcn  Expr=cos(u[1])*cos(u[2])
  9x1->3x3 : simulink/Math Operations/Reshape  OutputDimensionality=Customize  OutputDimensions=[3,3]
  Mux2 : Mux  Orientation=down  Inputs=9
  DCM : Outport
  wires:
  9x1->3x3/1 -> DCM/1
  11/1 -> Mux2/1
  21/1 -> Mux2/2
  31/1 -> Mux2/3
  rpw/1 -> 31/1, 21/1, 11/1, 32/1, 22/1, 12/1, 33/1, 23/1, 13/1
  12/1 -> Mux2/4
  22/1 -> Mux2/5
  32/1 -> Mux2/6
  Mux2/1 -> 9x1->3x3/1
  13/1 -> Mux2/7
  23/1 -> Mux2/8
  33/1 -> Mux2/9

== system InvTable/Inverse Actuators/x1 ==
  note: Auxiliary diagnostic output vector: 1: valve opening 2: C1 pressure 3: C2 pressure 4: delta pressure 5: force 6: velocity 7: C1 flow 8: C2 flow 9: total flow 10: kinematic flow 11: compressibility flow 12: leakage flow 13: iteration error
  note: Note: "1" and "2" denote actuator cylinders on either side of the actuator piston. With positive valve drive, oil is ported into cylinder 1, resulting in positive displacement.
  note: Parameter vector: 1: oil bulk modulus (force/displ^2) 2: servovalve natural frequency (Hz) 3: servovalve damping ratio 4: servovalve overlap 5: rated pressure (force/displ^2) 6: flow at rated pressure (displ^3/sec) 7: actuator piston area 1 (displ^2) 8: actuator piston area 2 (displ^2) 9: actuator usable stroke 1 (displ) 10: actuator usable stroke 2 (displ) 11: actuator end cushion length 1 (displ) 12: actuator end cushion length 2 (displ) 13: actuator parasitic damping factor 14: cross-chamber leakage factor (flow/press) 15: ratio port openings according to area 16: sample period (sec) Conversion factors used for converting signals from external (user) to internal (canonical) units: 17: displacement 18: velocity 19: force 20: pressure 21: flow Other: 22: delta-F feedback gain 23: inverse solver (0: exact, 1: approx)
  displ : Inport
  veloc : Inport  Port=2
  force : Inport  Port=3
  spl press : Inport  Port=4
  rtn press : Inport  Port=5
  abs : Abs
  invactuator : S-Function  FunctionName=invactuator  Parameters=params
  total flow sel : Selector  Elements=9  InputPortWidth=13
  cmd : Outport
  flow : Outport  Port=2
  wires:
  spl press/1 -> invactuator/4
  rtn press/1 -> invactuator/5
  displ/1 -> invactuator/1
  invactuator/1 -> cmd/1
  veloc/1 -> invactuator/2
  force/1 -> invactuator/3
  invactuator/2 -> total flow sel/1
  total flow sel/1 -> abs/1
  abs/1 -> flow/1

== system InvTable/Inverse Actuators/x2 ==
  note: Parameter vector: 1: oil bulk modulus (force/displ^2) 2: servovalve natural frequency (Hz) 3: servovalve damping ratio 4: servovalve overlap 5: rated pressure (force/displ^2) 6: flow at rated pressure (displ^3/sec) 7: actuator piston area 1 (displ^2) 8: actuator piston area 2 (displ^2) 9: actuator usable stroke 1 (displ) 10: actuator usable stroke 2 (displ) 11: actuator endcap length 1 (displ) 12: actuator endcap length 2 (displ) 13: actuator parasitic damping factor 14: cross-chamber leakage factor (flow/press) 15: ratio port openings according to area 16: sample period (sec) Conversion factors used for converting signals from external (user) to internal (canonical) units: 17: displacement 18: velocity 19: force 20: pressure 21: flow Other: 22: delta-F feedback gain 23: inverse solver (0: exact, 1: approx)
  note: Note: "1" and "2" denote actuator cylinders on either side of the actuator piston. With positive valve drive, oil is ported into cylinder 1, resulting in positive displacement.
  note: Auxiliary diagnostic output vector: 1: valve opening 2: C1 pressure 3: C2 pressure 4: delta pressure 5: force 6: velocity 7: C1 flow 8: C2 flow 9: total flow 10: kinematic flow 11: compressibility flow 12: leakage flow 13: iteration error
  displ : Inport
  veloc : Inport  Port=2
  force : Inport  Port=3
  spl press : Inport  Port=4
  rtn press : Inport  Port=5
  abs : Abs
  invactuator : S-Function  FunctionName=invactuator  Parameters=params
  total flow sel : Selector  Elements=9  InputPortWidth=13
  cmd : Outport
  flow : Outport  Port=2
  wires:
  abs/1 -> flow/1
  total flow sel/1 -> abs/1
  invactuator/2 -> total flow sel/1
  force/1 -> invactuator/3
  veloc/1 -> invactuator/2
  invactuator/1 -> cmd/1
  displ/1 -> invactuator/1
  rtn press/1 -> invactuator/5
  spl press/1 -> invactuator/4

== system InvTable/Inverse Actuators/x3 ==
  note: Auxiliary diagnostic output vector: 1: valve opening 2: C1 pressure 3: C2 pressure 4: delta pressure 5: force 6: velocity 7: C1 flow 8: C2 flow 9: total flow 10: kinematic flow 11: compressibility flow 12: leakage flow 13: iteration error
  note: Note: "1" and "2" denote actuator cylinders on either side of the actuator piston. With positive valve drive, oil is ported into cylinder 1, resulting in positive displacement.
  note: Parameter vector: 1: oil bulk modulus (force/displ^2) 2: servovalve natural frequency (Hz) 3: servovalve damping ratio 4: servovalve overlap 5: rated pressure (force/displ^2) 6: flow at rated pressure (displ^3/sec) 7: actuator piston area 1 (displ^2) 8: actuator piston area 2 (displ^2) 9: actuator usable stroke 1 (displ) 10: actuator usable stroke 2 (displ) 11: actuator end cushion length 1 (displ) 12: actuator end cushion length 2 (displ) 13: actuator parasitic damping factor 14: cross-chamber leakage factor (flow/press) 15: ratio port openings according to area 16: sample period (sec) Conversion factors used for converting signals from external (user) to internal (canonical) units: 17: displacement 18: velocity 19: force 20: pressure 21: flow Other: 22: delta-F feedback gain 23: inverse solver (0: exact, 1: approx)
  displ : Inport
  veloc : Inport  Port=2
  force : Inport  Port=3
  spl press : Inport  Port=4
  rtn press : Inport  Port=5
  abs : Abs
  invactuator : S-Function  FunctionName=invactuator  Parameters=params
  total flow sel : Selector  Elements=9  InputPortWidth=13
  cmd : Outport
  flow : Outport  Port=2
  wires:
  spl press/1 -> invactuator/4
  rtn press/1 -> invactuator/5
  displ/1 -> invactuator/1
  invactuator/1 -> cmd/1
  veloc/1 -> invactuator/2
  force/1 -> invactuator/3
  invactuator/2 -> total flow sel/1
  total flow sel/1 -> abs/1
  abs/1 -> flow/1

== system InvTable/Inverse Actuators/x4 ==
  note: Parameter vector: 1: oil bulk modulus (force/displ^2) 2: servovalve natural frequency (Hz) 3: servovalve damping ratio 4: servovalve overlap 5: rated pressure (force/displ^2) 6: flow at rated pressure (displ^3/sec) 7: actuator piston area 1 (displ^2) 8: actuator piston area 2 (displ^2) 9: actuator usable stroke 1 (displ) 10: actuator usable stroke 2 (displ) 11: actuator end cushion length 1 (displ) 12: actuator end cushion length 2 (displ) 13: actuator parasitic damping factor 14: cross-chamber leakage factor (flow/press) 15: ratio port openings according to area 16: sample period (sec) Conversion factors used for converting signals from external (user) to internal (canonical) units: 17: displacement 18: velocity 19: force 20: pressure 21: flow Other: 22: delta-F feedback gain 23: inverse solver (0: exact, 1: approx)
  note: Note: "1" and "2" denote actuator cylinders on either side of the actuator piston. With positive valve drive, oil is ported into cylinder 1, resulting in positive displacement.
  note: Auxiliary diagnostic output vector: 1: valve opening 2: C1 pressure 3: C2 pressure 4: delta pressure 5: force 6: velocity 7: C1 flow 8: C2 flow 9: total flow 10: kinematic flow 11: compressibility flow 12: leakage flow 13: iteration error
  displ : Inport
  veloc : Inport  Port=2
  force : Inport  Port=3
  spl press : Inport  Port=4
  rtn press : Inport  Port=5
  abs : Abs
  invactuator : S-Function  FunctionName=invactuator  Parameters=params
  total flow sel : Selector  Elements=9  InputPortWidth=13
  cmd : Outport
  flow : Outport  Port=2
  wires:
  abs/1 -> flow/1
  total flow sel/1 -> abs/1
  invactuator/2 -> total flow sel/1
  force/1 -> invactuator/3
  veloc/1 -> invactuator/2
  invactuator/1 -> cmd/1
  displ/1 -> invactuator/1
  rtn press/1 -> invactuator/5
  spl press/1 -> invactuator/4

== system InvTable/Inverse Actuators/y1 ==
  note: Auxiliary diagnostic output vector: 1: valve opening 2: C1 pressure 3: C2 pressure 4: delta pressure 5: force 6: velocity 7: C1 flow 8: C2 flow 9: total flow 10: kinematic flow 11: compressibility flow 12: leakage flow 13: iteration error
  note: Note: "1" and "2" denote actuator cylinders on either side of the actuator piston. With positive valve drive, oil is ported into cylinder 1, resulting in positive displacement.
  note: Parameter vector: 1: oil bulk modulus (force/displ^2) 2: servovalve natural frequency (Hz) 3: servovalve damping ratio 4: servovalve overlap 5: rated pressure (force/displ^2) 6: flow at rated pressure (displ^3/sec) 7: actuator piston area 1 (displ^2) 8: actuator piston area 2 (displ^2) 9: actuator usable stroke 1 (displ) 10: actuator usable stroke 2 (displ) 11: actuator end cushion length 1 (displ) 12: actuator end cushion length 2 (displ) 13: actuator parasitic damping factor 14: cross-chamber leakage factor (flow/press) 15: ratio port openings according to area 16: sample period (sec) Conversion factors used for converting signals from external (user) to internal (canonical) units: 17: displacement 18: velocity 19: force 20: pressure 21: flow Other: 22: delta-F feedback gain 23: inverse solver (0: exact, 1: approx)
  displ : Inport
  veloc : Inport  Port=2
  force : Inport  Port=3
  spl press : Inport  Port=4
  rtn press : Inport  Port=5
  abs : Abs
  invactuator : S-Function  FunctionName=invactuator  Parameters=params
  total flow sel : Selector  Elements=9  InputPortWidth=13
  cmd : Outport
  flow : Outport  Port=2
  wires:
  spl press/1 -> invactuator/4
  rtn press/1 -> invactuator/5
  displ/1 -> invactuator/1
  invactuator/1 -> cmd/1
  veloc/1 -> invactuator/2
  force/1 -> invactuator/3
  invactuator/2 -> total flow sel/1
  total flow sel/1 -> abs/1
  abs/1 -> flow/1

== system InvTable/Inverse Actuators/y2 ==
  note: Parameter vector: 1: oil bulk modulus (force/displ^2) 2: servovalve natural frequency (Hz) 3: servovalve damping ratio 4: servovalve overlap 5: rated pressure (force/displ^2) 6: flow at rated pressure (displ^3/sec) 7: actuator piston area 1 (displ^2) 8: actuator piston area 2 (displ^2) 9: actuator usable stroke 1 (displ) 10: actuator usable stroke 2 (displ) 11: actuator end cushion length 1 (displ) 12: actuator end cushion length 2 (displ) 13: actuator parasitic damping factor 14: cross-chamber leakage factor (flow/press) 15: ratio port openings according to area 16: sample period (sec) Conversion factors used for converting signals from external (user) to internal (canonical) units: 17: displacement 18: velocity 19: force 20: pressure 21: flow Other: 22: delta-F feedback gain 23: inverse solver (0: exact, 1: approx)
  note: Note: "1" and "2" denote actuator cylinders on either side of the actuator piston. With positive valve drive, oil is ported into cylinder 1, resulting in positive displacement.
  note: Auxiliary diagnostic output vector: 1: valve opening 2: C1 pressure 3: C2 pressure 4: delta pressure 5: force 6: velocity 7: C1 flow 8: C2 flow 9: total flow 10: kinematic flow 11: compressibility flow 12: leakage flow 13: iteration error
  displ : Inport
  veloc : Inport  Port=2
  force : Inport  Port=3
  spl press : Inport  Port=4
  rtn press : Inport  Port=5
  abs : Abs
  invactuator : S-Function  FunctionName=invactuator  Parameters=params
  total flow sel : Selector  Elements=9  InputPortWidth=13
  cmd : Outport
  flow : Outport  Port=2
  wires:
  abs/1 -> flow/1
  total flow sel/1 -> abs/1
  invactuator/2 -> total flow sel/1
  force/1 -> invactuator/3
  veloc/1 -> invactuator/2
  invactuator/1 -> cmd/1
  displ/1 -> invactuator/1
  rtn press/1 -> invactuator/5
  spl press/1 -> invactuator/4

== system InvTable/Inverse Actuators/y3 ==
  note: Auxiliary diagnostic output vector: 1: valve opening 2: C1 pressure 3: C2 pressure 4: delta pressure 5: force 6: velocity 7: C1 flow 8: C2 flow 9: total flow 10: kinematic flow 11: compressibility flow 12: leakage flow 13: iteration error
  note: Note: "1" and "2" denote actuator cylinders on either side of the actuator piston. With positive valve drive, oil is ported into cylinder 1, resulting in positive displacement.
  note: Parameter vector: 1: oil bulk modulus (force/displ^2) 2: servovalve natural frequency (Hz) 3: servovalve damping ratio 4: servovalve overlap 5: rated pressure (force/displ^2) 6: flow at rated pressure (displ^3/sec) 7: actuator piston area 1 (displ^2) 8: actuator piston area 2 (displ^2) 9: actuator usable stroke 1 (displ) 10: actuator usable stroke 2 (displ) 11: actuator end cushion length 1 (displ) 12: actuator end cushion length 2 (displ) 13: actuator parasitic damping factor 14: cross-chamber leakage factor (flow/press) 15: ratio port openings according to area 16: sample period (sec) Conversion factors used for converting signals from external (user) to internal (canonical) units: 17: displacement 18: velocity 19: force 20: pressure 21: flow Other: 22: delta-F feedback gain 23: inverse solver (0: exact, 1: approx)
  displ : Inport
  veloc : Inport  Port=2
  force : Inport  Port=3
  spl press : Inport  Port=4
  rtn press : Inport  Port=5
  abs : Abs
  invactuator : S-Function  FunctionName=invactuator  Parameters=params
  total flow sel : Selector  Elements=9  InputPortWidth=13
  cmd : Outport
  flow : Outport  Port=2
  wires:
  spl press/1 -> invactuator/4
  rtn press/1 -> invactuator/5
  displ/1 -> invactuator/1
  invactuator/1 -> cmd/1
  veloc/1 -> invactuator/2
  force/1 -> invactuator/3
  invactuator/2 -> total flow sel/1
  total flow sel/1 -> abs/1
  abs/1 -> flow/1

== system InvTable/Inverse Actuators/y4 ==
  note: Parameter vector: 1: oil bulk modulus (force/displ^2) 2: servovalve natural frequency (Hz) 3: servovalve damping ratio 4: servovalve overlap 5: rated pressure (force/displ^2) 6: flow at rated pressure (displ^3/sec) 7: actuator piston area 1 (displ^2) 8: actuator piston area 2 (displ^2) 9: actuator usable stroke 1 (displ) 10: actuator usable stroke 2 (displ) 11: actuator end cushion length 1 (displ) 12: actuator end cushion length 2 (displ) 13: actuator parasitic damping factor 14: cross-chamber leakage factor (flow/press) 15: ratio port openings according to area 16: sample period (sec) Conversion factors used for converting signals from external (user) to internal (canonical) units: 17: displacement 18: velocity 19: force 20: pressure 21: flow Other: 22: delta-F feedback gain 23: inverse solver (0: exact, 1: approx)
  note: Note: "1" and "2" denote actuator cylinders on either side of the actuator piston. With positive valve drive, oil is ported into cylinder 1, resulting in positive displacement.
  note: Auxiliary diagnostic output vector: 1: valve opening 2: C1 pressure 3: C2 pressure 4: delta pressure 5: force 6: velocity 7: C1 flow 8: C2 flow 9: total flow 10: kinematic flow 11: compressibility flow 12: leakage flow 13: iteration error
  displ : Inport
  veloc : Inport  Port=2
  force : Inport  Port=3
  spl press : Inport  Port=4
  rtn press : Inport  Port=5
  abs : Abs
  invactuator : S-Function  FunctionName=invactuator  Parameters=params
  total flow sel : Selector  Elements=9  InputPortWidth=13
  cmd : Outport
  flow : Outport  Port=2
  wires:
  abs/1 -> flow/1
  total flow sel/1 -> abs/1
  invactuator/2 -> total flow sel/1
  force/1 -> invactuator/3
  veloc/1 -> invactuator/2
  invactuator/1 -> cmd/1
  displ/1 -> invactuator/1
  rtn press/1 -> invactuator/5
  spl press/1 -> invactuator/4

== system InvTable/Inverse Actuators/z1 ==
  note: Auxiliary diagnostic output vector: 1: valve opening 2: C1 pressure 3: C2 pressure 4: delta pressure 5: force 6: velocity 7: C1 flow 8: C2 flow 9: total flow 10: kinematic flow 11: compressibility flow 12: leakage flow 13: iteration error
  note: Note: "1" and "2" denote actuator cylinders on either side of the actuator piston. With positive valve drive, oil is ported into cylinder 1, resulting in positive displacement.
  note: Parameter vector: 1: oil bulk modulus (force/displ^2) 2: servovalve natural frequency (Hz) 3: servovalve damping ratio 4: servovalve overlap 5: rated pressure (force/displ^2) 6: flow at rated pressure (displ^3/sec) 7: actuator piston area 1 (displ^2) 8: actuator piston area 2 (displ^2) 9: actuator usable stroke 1 (displ) 10: actuator usable stroke 2 (displ) 11: actuator end cushion length 1 (displ) 12: actuator end cushion length 2 (displ) 13: actuator parasitic damping factor 14: cross-chamber leakage factor (flow/press) 15: ratio port openings according to area 16: sample period (sec) Conversion factors used for converting signals from external (user) to internal (canonical) units: 17: displacement 18: velocity 19: force 20: pressure 21: flow Other: 22: delta-F feedback gain 23: inverse solver (0: exact, 1: approx)
  displ : Inport
  veloc : Inport  Port=2
  force : Inport  Port=3
  spl press : Inport  Port=4
  rtn press : Inport  Port=5
  abs : Abs
  invactuator : S-Function  FunctionName=invactuator  Parameters=params
  total flow sel : Selector  Elements=9  InputPortWidth=13
  cmd : Outport
  flow : Outport  Port=2
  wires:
  spl press/1 -> invactuator/4
  rtn press/1 -> invactuator/5
  displ/1 -> invactuator/1
  invactuator/1 -> cmd/1
  veloc/1 -> invactuator/2
  force/1 -> invactuator/3
  invactuator/2 -> total flow sel/1
  total flow sel/1 -> abs/1
  abs/1 -> flow/1
